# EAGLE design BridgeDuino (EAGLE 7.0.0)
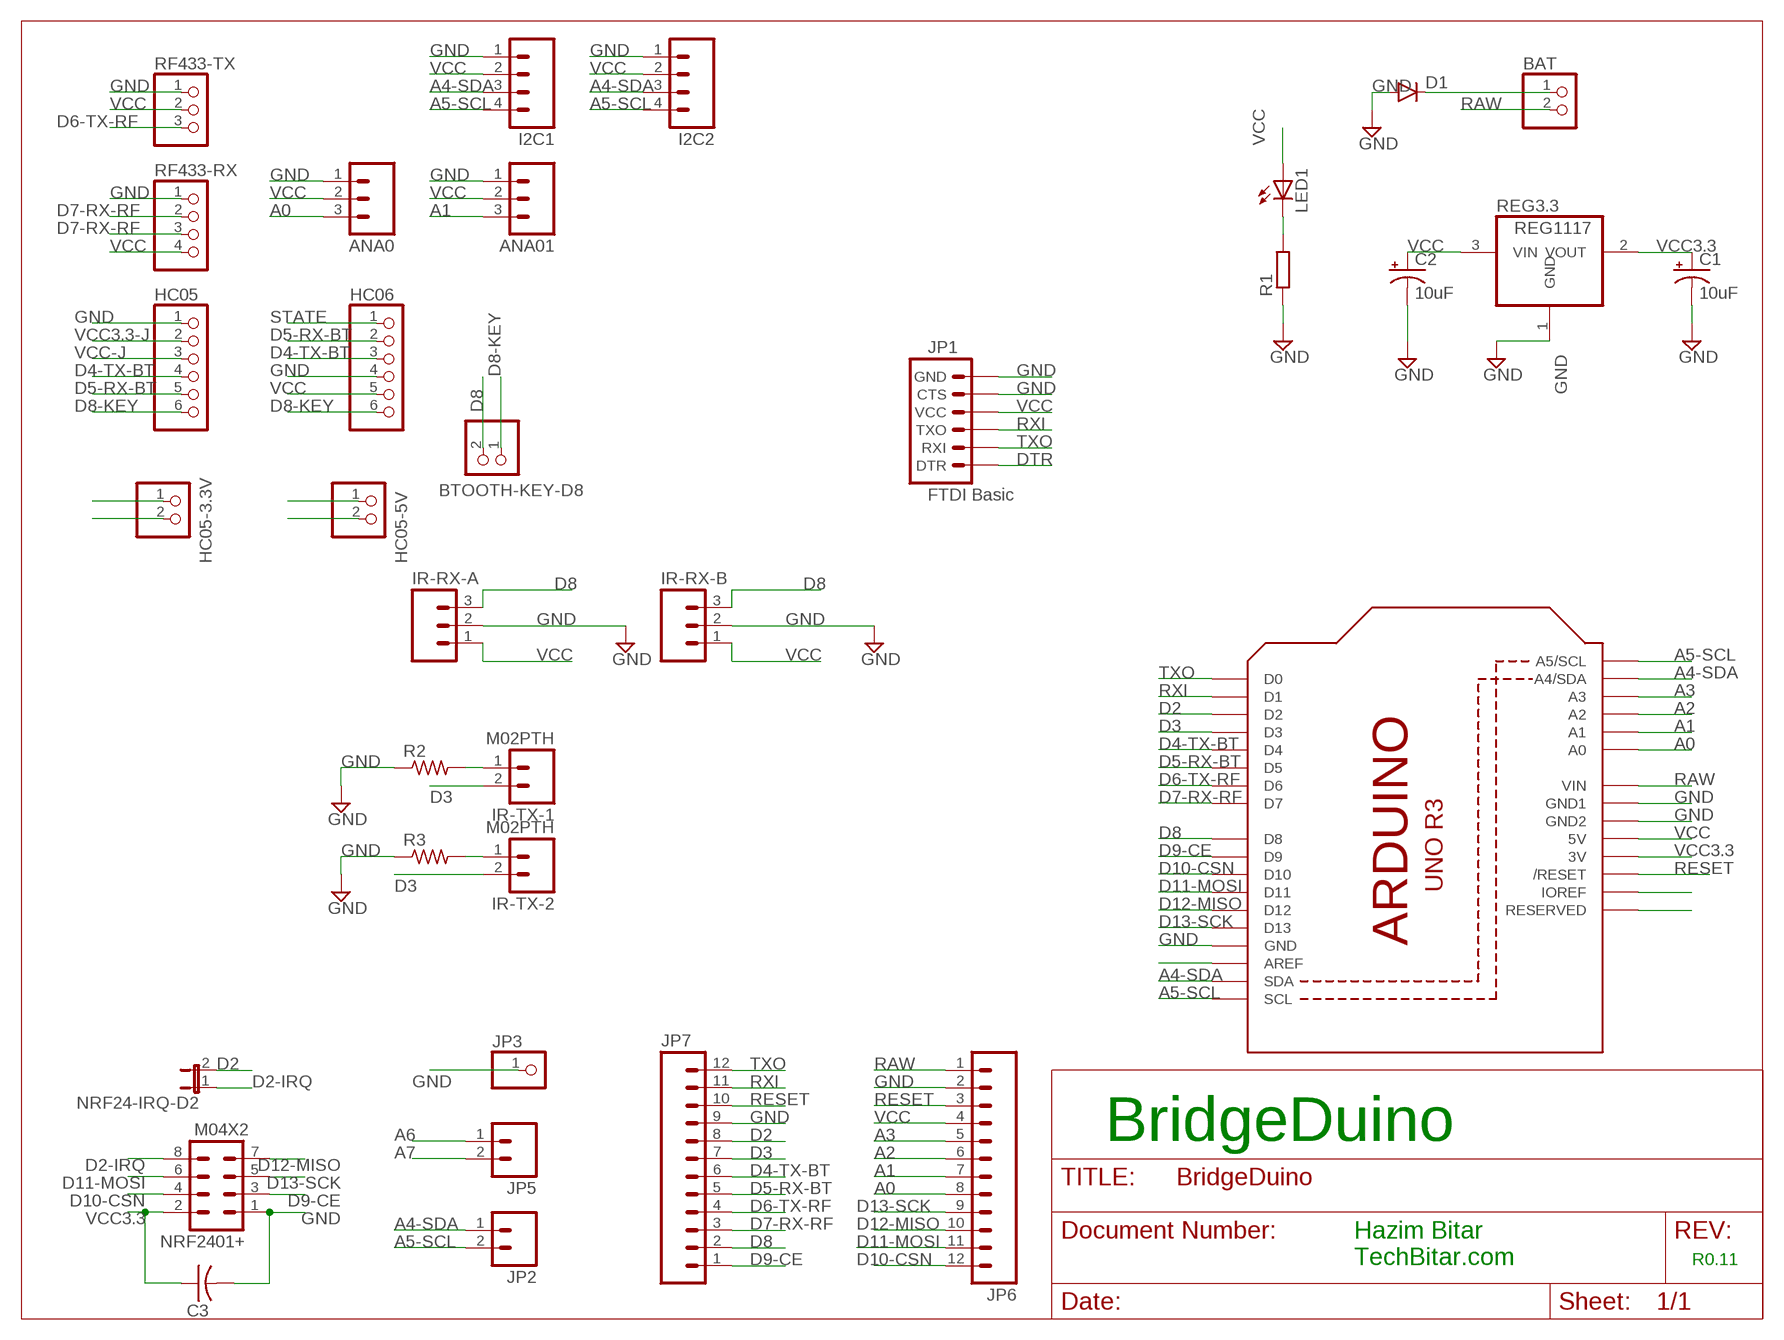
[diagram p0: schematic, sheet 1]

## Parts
ANA0  M03PTH  [1X03]
ANA01  M03PTH  [1X03]
BAT  PINHD-1X2  [1X02]
BTOOTH-KEY-D8  PINHD-1X2  [1X02]
C1  10uF  10UF-16V-10%(TANT)  [EIA3216]
C2  10uF  10UF-16V-10%(TANT)  [EIA3216]
C3  C-US025-024X044  [C025-024X044]
D1  DIODE  [DIODE-1N4001-KIT]
HC05  PINHD-1X6  [1X06]
HC05-3.3V  PINHD-1X2  [1X02]
HC05-5V  PINHD-1X2  [1X02]
HC06  PINHD-1X6  [1X06]
I2C1  M04PTH  [1X04]
I2C2  M04PTH  [1X04]
IR-RX-A  M03PTH  [1X03]
IR-RX-B  M03PTH  [1X03]
IR-TX-1  M02PTH  [1X02]
IR-TX-2  M02PTH  [1X02]
JP1  FTDI Basic  ARDUINO_SERIAL_PROGRAMPTH  [1X06]
JP2  M02PTH  [1X02]
JP3  PINHD-1X1  [1X01]
JP5  M02PTH  [1X02]
JP6  M12PTH  [1X12]
JP7  M12PTH  [1X12]
LED1  LED3MM  [LED3MM]
NRF24-IRQ-D2  JUMPER-2PTH  [1X02]
NRF2401+  M04X2  [2X4]
R1  R-EU_0204/5  [0204/5]
R2  R-US_0204/2V  [0204V]
R3  R-US_0204/2V  [0204V]
REG3.3  REG1117  [SOT223]
RF433-RX  PINHD-1X4  [1X04]
RF433-TX  PINHD-1X3  [1X03]
U1  ARDUINOR3-DIMENSION  [ARDUINOR3]

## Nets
A0 [vcc]: ANA0.3 JP6.8 U1.A0
A1 [vcc]: ANA01.3 JP6.7 U1.A1
A2 [vcc]: JP6.6 U1.A2
A3 [vcc]: JP6.5 U1.A3
A4-SDA [vcc]: I2C1.3 I2C2.3 JP2.1 U1.A4(A4/SDA) U1.SDA
A5-SCL [vcc]: I2C1.4 I2C2.4 JP2.2 U1.A5(A5/SCL) U1.SCL
A6 [vcc]: JP5.1
A7 [vcc]: JP5.2
D2 [vcc]: JP7.8 NRF24-IRQ-D2.2 U1.D2
D2-IRQ [vcc]: NRF24-IRQ-D2.1 NRF2401+.8
D3 [vcc]: IR-TX-1.2 IR-TX-2.2 JP7.7 U1.D3
D4-TX-BT [vcc]: HC05.4 HC06.3 JP7.6 U1.D4
D5-RX-BT [vcc]: HC05.5 HC06.2 JP7.5 U1.D5
D6-TX-RF [vcc]: JP7.4 RF433-TX.3 U1.D6
D7-RX-RF [vcc]: JP7.3 RF433-RX.2 RF433-RX.3 U1.D7
D8 [vcc]: BTOOTH-KEY-D8.2 IR-RX-A.3 IR-RX-B.3 JP7.2 U1.D8
D8-KEY [vcc]: BTOOTH-KEY-D8.1 HC05.6 HC06.6
D9-CE [vcc]: JP7.1 NRF2401+.3 U1.D9
D10-CSN [vcc]: JP6.12 NRF2401+.4 U1.D10
D11-MOSI: JP6.11 NRF2401+.6 U1.D11
D12-MISO [vcc]: JP6.10 NRF2401+.7 U1.D12
D13-SCK [vcc]: JP6.9 NRF2401+.5 U1.D13
DTR: JP1.1(DTR)
GND [vcc]: ANA0.1 ANA01.1 C1.C(-) C2.C(-) C3.2 D1.A HC05.1 HC06.4 I2C1.1 I2C2.1 IR-RX-A.2 IR-RX-B.2 JP1.5(CTS) JP1.6(GND) JP3.1 JP6.2 JP7.9 NRF2401+.1 R1.1 R2.1 R3.1 REG3.3.1(GND) RF433-RX.1 RF433-TX.1 U1.GND U1.GND1 U1.GND2
N$1: BAT.1 D1.C
N$2: IR-TX-2.1 R3.2
N$3: LED1.K(C) R1.2
N$4: IR-TX-1.1 R2.2
N$7 [vcc]: U1.IOREF
N$8 [vcc]: U1.RESERVED
N$24 [vcc]: U1.AREF
RAW [vcc]: BAT.2 JP6.1 U1.VIN
RESET [vcc]: JP6.3 JP7.10 U1.RESET(/RESET)
RXI [vcc]: JP1.3(TXO) JP7.11 U1.D1
STATE [vcc]: HC06.1
TXO [vcc]: JP1.2(RXI) JP7.12 U1.D0
VCC [vcc]: ANA0.2 ANA01.2 C2.A(+) HC05-5V.2 HC06.5 I2C1.2 I2C2.2 IR-RX-A.1 IR-RX-B.1 JP1.4(VCC) JP6.4 LED1.A REG3.3.3(VIN) RF433-RX.4 RF433-TX.2 U1.5V
VCC3.3 [vcc]: C1.A(+) C3.1 HC05-3.3V.2 NRF2401+.2 REG3.3.2(VOUT) U1.3V
VCC3.3-J [vcc]: HC05-3.3V.1 HC05.2
VCC-J [vcc]: HC05-5V.1 HC05.3

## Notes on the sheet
- BridgeDuino
- Hazim Bitar
  TechBitar.com
- R0.11

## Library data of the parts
ANA0 ANA01 IR-RX-A IR-RX-B = SparkFun-Connectors:M03: Header 3 Standard 3-pin 0.1" header. Use with straight break away headers (SKU : PRT-00116), right angle break away headers (PRT-00553), swiss pins (PRT-00743), machine pins (PRT-00117), and female headers (PRT-00115). Molex polarized connector foot print use with SKU : PRT-08232 with associated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
BAT BTOOTH-KEY-D8 HC05-3.3V HC05-5V = pinhead:PINHD-1X2: PIN HEADER
C1 C2 = SparkFun-Capacitors:10UF-16V-10%(TANT): CAP-00811; PROD_ID: CAP-00811
C3 = adafruit:C-US: CAPACITOR, American symbol
D1 = SparkFun-DiscreteSemi:DIODE: Diode
HC05 HC06 = adafruit:PINHD-1X6: PIN HEADER
I2C1 I2C2 = SparkFun-Connectors:M04: Header 4 Standard 4-pin 0.1" header. Use with straight break away headers (SKU : PRT-00116), right angle break away headers (PRT-00553), swiss pins (PRT-00743), machine pins (PRT-00117), and female headers (PRT-00115). Molex polarized connector foot print use with SKU : PRT-08231 with associated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
IR-TX-1 IR-TX-2 = SparkFun-Connectors:M02: Standard 2-pin 0.1" header. Use with
JP1 = SparkFun:ARDUINO_SERIAL_PROGRAM
JP2 JP5 = SparkFun:M02: Header 2
JP3 = adafruit:PINHD-1X1: Pin header 1x1 for 0.1" spacing
JP6 JP7 = SparkFun:M12: Header 12 Standard 12-pin 0.1" header. Use with straight break away headers (SKU : PRT-00116), right angle break away headers (PRT-00553), swiss pins (PRT-00743), machine pins (PRT-00117), and female headers (PRT-00115).
LED1 = led:LED: LED
NRF24-IRQ-D2 = SparkFun-Retired:JUMPER-2: Jumper
NRF2401+ = SparkFun-Connectors:M04X2: .1" header, two rows of four.
R1 = resistor:R-EU_: RESISTOR, European symbol
R2 R3 = adafruit:R-US_: RESISTOR, American symbol
REG3.3 = burr-brown:REG1117: 800mA and 1A Low Dropout (LDO) Positive Regulator 1.8V, 2.5V, 2.85V, 3.3V, 5V, and Adj; MPN: REG1117; OC_FARNELL: 1097566; OC_NEWARK: 14P6981
RF433-RX = pinhead:PINHD-1X4: PIN HEADER
RF433-TX = pinhead:PINHD-1X3: PIN HEADER
U1 = adafruit:ARDUINOR3: This is a new object for the new Arduino R3 - with extra pins that you may want to use (such as IOref, and duplicated A4/A5

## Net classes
0 default: width 0.203 mm
1 vcc: width 0.203 mm

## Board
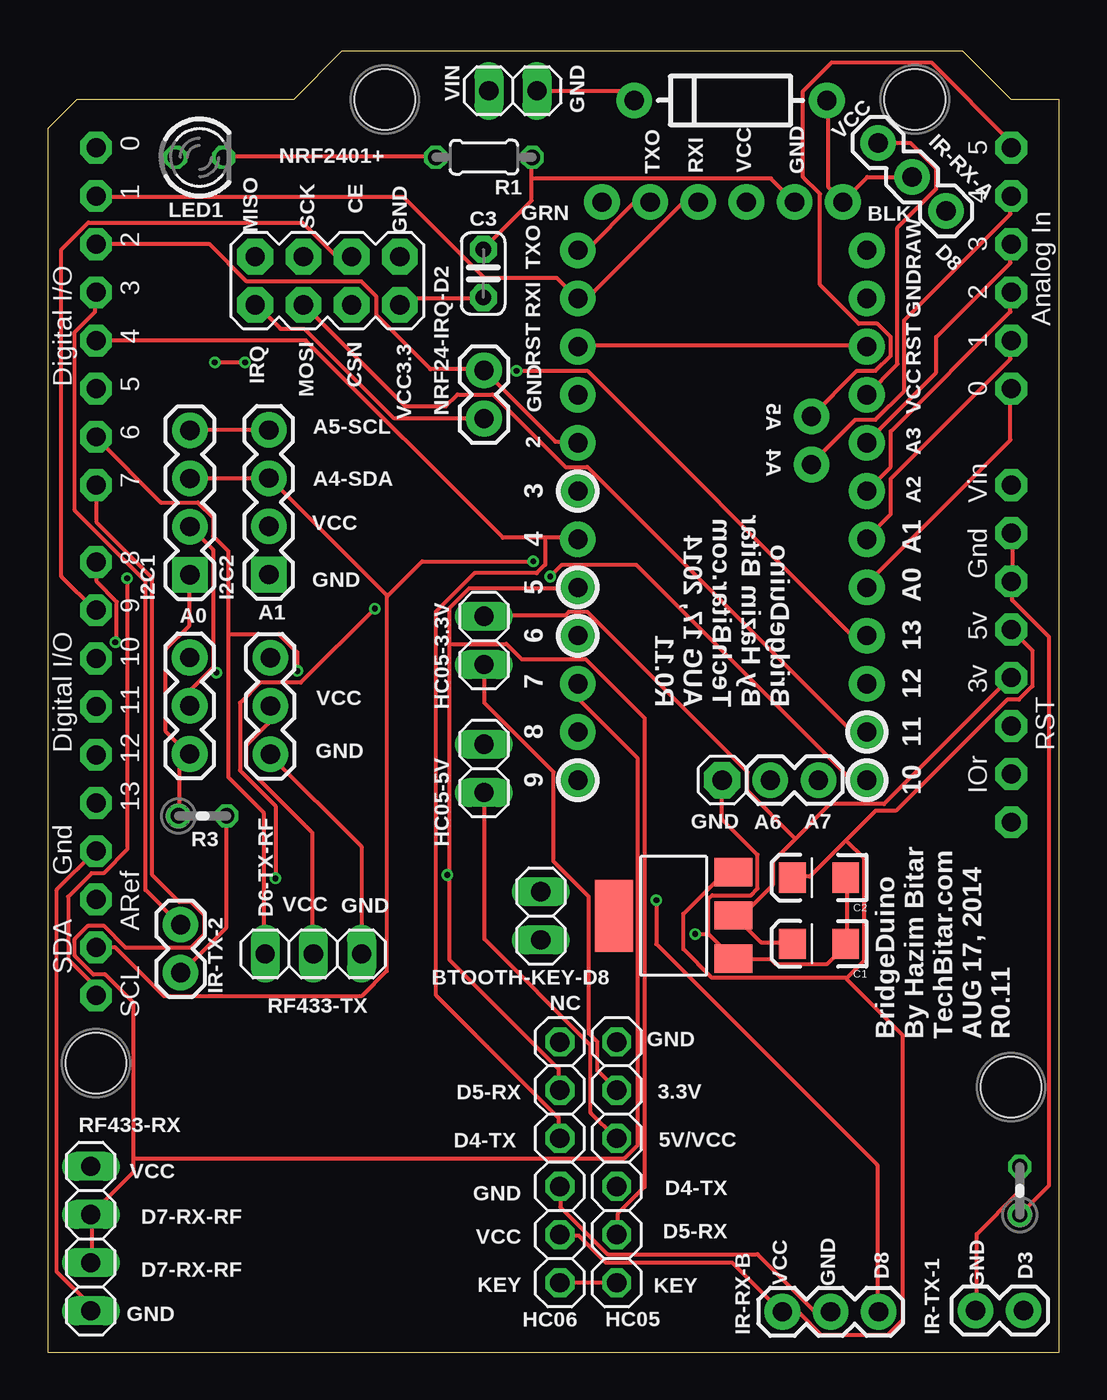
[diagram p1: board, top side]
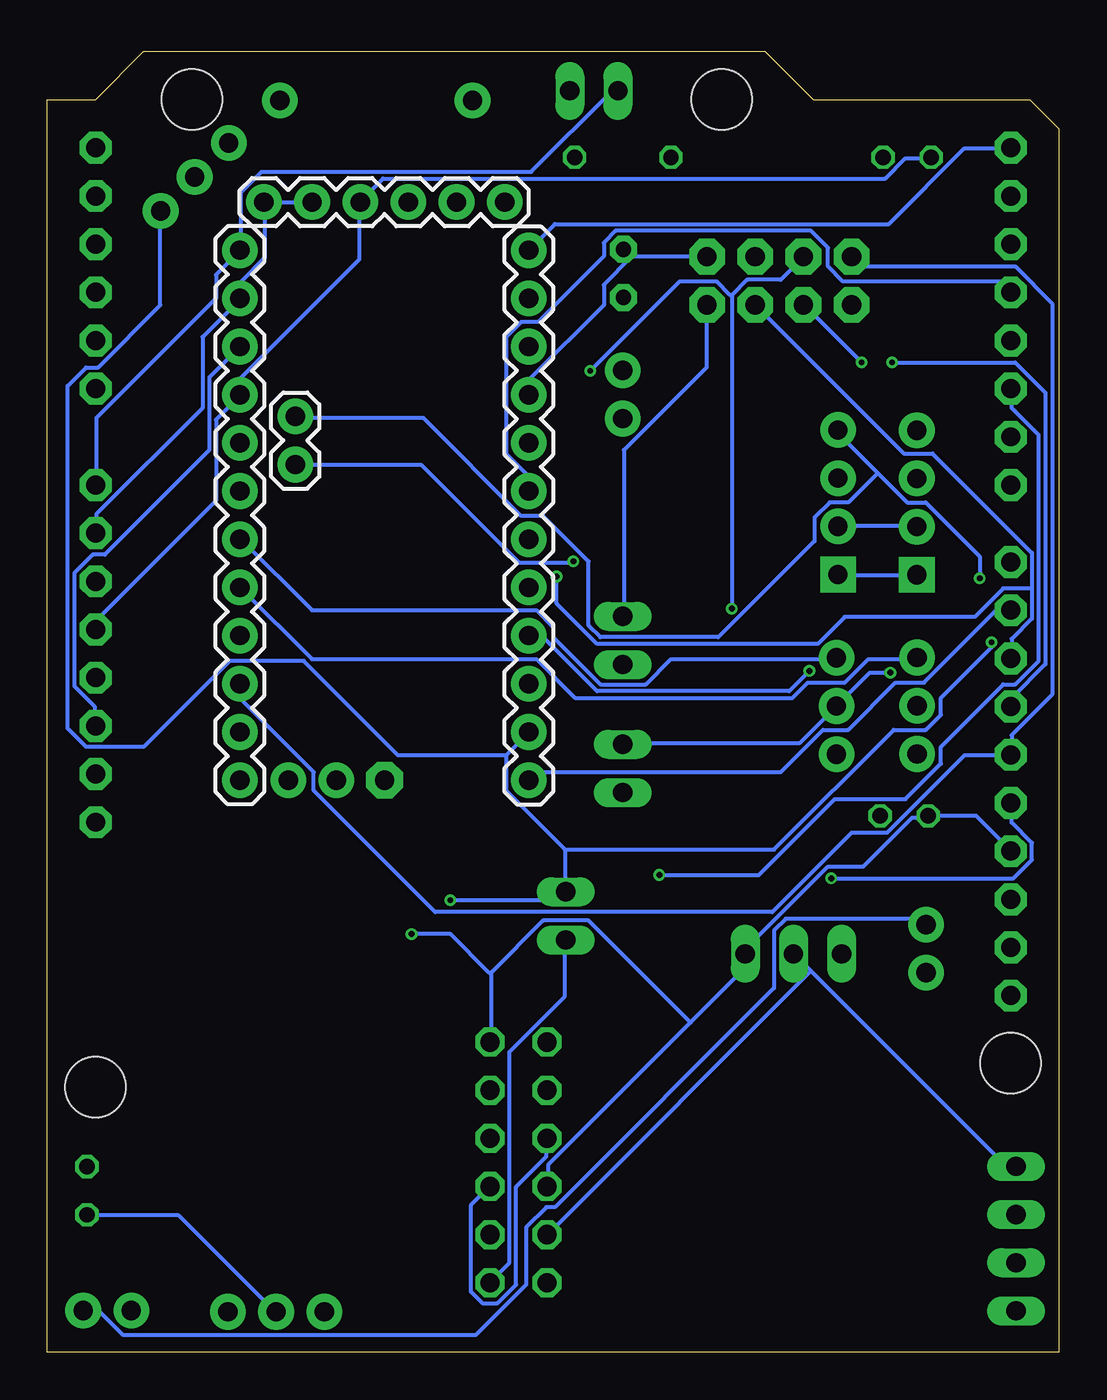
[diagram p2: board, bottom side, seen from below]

Size 53.34 x 68.58 mm. Coordinates in mm from the lower left corner, seen from the top.
Copper layers (1*2*15*16): Top 0.035mm / dielectric 0.2mm / Route2 0.0175mm / dielectric 1.1mm / Route15 0.0175mm / dielectric 0.2mm / Bottom 0.035mm
Design rules "SeeedStudio_DRU_no_angle_20130527 *": minimum track width 6mil, minimum drill 12mil, track to track 6mil, track to pad 6mil, pad to pad 6mil, via to via 6mil, smd to smd 0mil, copper to edge 10mil, drill to drill 10mil, minimum pad ring 6mil, minimum via ring 6mil, stop-mask expansion 2mil, vias tented up to drill 25mil, thermal gap 10mil
Holes 3.2 mm at 2.54,15.24 17.78,66.04 45.72,66.04 50.8,13.97

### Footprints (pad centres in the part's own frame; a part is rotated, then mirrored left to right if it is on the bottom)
1X03 = drill 1.016 pad 1.88: 1 0,0; 2 2.54,0; 3 5.08,0
1X02 = drill 1.016 long: 1 -1.27,0; 2 1.27,0
EIA3216 = smd 1.4 x 1.6: A 1.4,0; C -1.4,0
C025-024X044 = drill 0.813 pad 1.422 octagon: 1 -1.27,0; 2 1.27,0
DIODE-1N4001-KIT = drill 1.016 pad 1.88: A -5.08,0; C 5.08,0
1X06 = drill 1.016 octagon: 1 -6.35,0; 2 -3.81,0; 3 -1.27,0; 4 1.27,0; 5 3.81,0; 6 6.35,0
1X04 = drill 1.016 pad 1.88 square: 1 0,0 | drill 1.016 pad 1.88: 2 2.54,0; 3 5.08,0; 4 7.62,0
1X02' = drill 1.016 pad 1.88: 1 0,0; 2 2.54,0
1X06' = drill 1.016 pad 1.88: 1 0,0; 2 2.54,0; 3 5.08,0; 4 7.62,0; 5 10.16,0; 6 12.7,0
1X01 = drill 1.016 pad 1.93 octagon: 1 0,0
1X12 = drill 1.016 pad 1.88: 1 0,0; 2 2.54,0; 3 5.08,0; 4 7.62,0; 5 10.16,0; 6 12.7,0; 7 15.24,0; 8 17.78,0; 9 20.32,0; 10 22.86,0; 11 25.4,0; 12 27.94,0
LED3MM = drill 0.813 octagon: A -1.27,0; K 1.27,0
2X4 = drill 1.016 pad 1.88 octagon: 1 -3.81,-1.27; 2 -3.81,1.27; 3 -1.27,-1.27; 4 -1.27,1.27; 5 1.27,-1.27; 6 1.27,1.27; 7 3.81,-1.27; 8 3.81,1.27
0204/5 = drill 0.813 octagon: 1 -2.54,0; 2 2.54,0
0204V = drill 0.813 octagon: 1 -1.27,0; 2 1.27,0
SOT223 = smd 1.499 x 2.007: 1 -2.261,-3.15; 2 0.025,-3.15; 3 2.311,-3.15 | smd 3.81 x 2.007: 4 0,3.15
1X04' = drill 1.016 long: 1 -3.81,0; 2 -1.27,0; 3 1.27,0; 4 3.81,0
1X03' = drill 1.016 long: 1 -2.54,0; 2 0,0; 3 2.54,0
ARDUINOR3 = drill 1 pad 1.676 octagon: 3V 35.56,2.54; 5V 38.1,2.54; A0 50.8,2.54; A1 53.34,2.54; A2 55.88,2.54; A3 58.42,2.54; A4 60.96,2.54; A5 63.5,2.54; AREF 23.876,50.8; D0 63.5,50.8; D1 60.96,50.8; D2 58.42,50.8; D3 55.88,50.8; D4 53.34,50.8; D5 50.8,50.8; D6 48.26,50.8; D7 45.72,50.8; D8 41.656,50.8; D9 39.116,50.8; D10 36.576,50.8; D11 34.036,50.8; D12 31.496,50.8; D13 28.956,50.8; GND 26.416,50.8; GND1 43.18,2.54; GND2 40.64,2.54; IOREF 30.48,2.54; RESERVED 27.94,2.54; RESET 33.02,2.54; SCL 18.796,50.8; SDA 21.336,50.8; VIN 45.72,2.54

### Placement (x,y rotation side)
ANA0  7.48,31.54 90 top
ANA01  11.73,31.52 90 top
BAT  24.52,66.51 180 top
BTOOTH-KEY-D8  26,23 90 top
C1  40.66,21.52 180 top
C2  40.66,25.02 180 top
C3  22.96,56.87 90 top
D1  36,66 180 top
HC05  30,10 270 top
HC05-3.3V  23,37.52 90 top
HC05-5V  23,30.78 90 top
HC06  27,10 270 top
I2C1  7.49,40.98 90 top
I2C2  11.65,41 90 top
IR-RX-A  43.78,63.76 315 top
IR-RX-B  38.74,2.13 0 top
IR-TX-1  M02PTH  [1X02']  48.92,2.19 0 top
IR-TX-2  M02PTH  [1X02']  7,20 90 top
JP1  FTDI Basic  [1X06']  29.22,60.64 180 bottom
JP2  [1X02']  40.27,46.8 90 bottom
JP3  35.56,30.16 0 top
JP5  [1X02']  38.1,30.16 0 top
JP6  43.19,58.1 270 bottom
JP7  27.95,30.16 90 bottom
LED1  8,63 0 top
NRF24-IRQ-D2  [1X02']  23,49.22 90 top
NRF2401+  14.75,56.49 180 top
R1  23,63 180 top
R2  51.25,8.51 90 top
R3  8.16,28.27 0 top
REG3.3  33,23 90 top
RF433-RX  [1X04']  2.26,5.98 90 top
RF433-TX  [1X03']  14,21 180 top
U1  53.34,0 90 top

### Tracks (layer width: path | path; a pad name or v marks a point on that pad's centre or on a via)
A0
  Top 0.203: U1.A0 50.76,50.76 50.76,48.09 43.2,40.54 43.2,40.36 JP6.8
  Bottom 0.203: ANA0.3 7.56,36.54 10.05,36.54 11.29,35.29 13.25,35.29 14.05,34.49 25.51,34.49 27.56,36.54 39.38,36.54 43.12,40.27 JP6.8
A1
  Top 0.203: U1.A1 50.76,53.34 50.76,52.36 44.45,46.05 44.45,44.18 43.2,42.94 JP6.7
  Bottom 0.203: ANA01.3 11.73,36.54 20.45,36.54 21.78,35.2 24.18,35.2 26.67,37.69 26.67,38.23 27.56,39.12 39.38,39.12 43.12,42.85 JP6.7
A2
  Top 0.203: U1.A2 50.76,55.83 50.76,54.85 44.45,48.54 44.45,46.67 43.2,45.43 JP6.6
A3
  Top 0.203: U1.A3 50.76,58.41 50.76,57.43 46.85,53.52 46.85,51.65 43.2,48.01 JP6.5
A4-SDA  (via drill 0.3)
  Top 0.203: U1.A4 50.76,60.9 50.76,60.01 45.16,54.41 45.16,50.67 43.65,49.16 42.58,49.16 40.27,46.85 JP2.1 | U1.SDA 3.56,21.34 6.13,18.76 16.54,18.76 17.87,20.09 17.87,39.92 | 17.87,39.92 11.73,46.05 I2C2.3 11.56,46.05 7.56,46.05 I2C1.3 | v25.6,41.69 19.74,41.69 17.96,39.92 17.87,39.92
  Bottom 0.203: v25.6,41.69 25.69,41.6 28.45,41.6 33.6,46.76 40.18,46.76 JP2.1
A5-SCL  (via drill 0.3)
  Top 0.203: U1.A5 50.76,63.56 50.76,63.83 46.58,68.01 41.34,68.01 39.83,66.5 39.83,61.96 40.72,61.07 40.72,56.27 42.76,54.23 43.74,54.23 44.45,53.52 44.45,52.54 43.65,51.74 42.67,51.74 JP2.2 | v4.18,40.8 4.18,26.49 2.93,25.25 2.31,25.25 1.07,24 1.07,20.71 2.49,19.29 2.49,18.85 U1.SCL | I2C1.4 7.56,48.63 I2C2.4
  Bottom 0.203: v4.18,40.8 4.18,41.96 7.02,44.81 8,44.81 9.56,46.36 | 9.56,46.36 11.73,48.54 I2C2.4 | 9.56,46.36 11.11,44.81 12.09,44.81 12.89,44.01 12.89,42.76 17.96,37.69 24.18,37.69 24.8,38.32 24.8,41.69 27.2,44.09 28.36,44.09 33.52,49.25 40.18,49.25 JP2.2
D2
  Top 0.203: U1.D2 2.58,58.41 8.53,58.41 10.49,56.45 16.54,56.45 17.34,55.65 17.34,54.67 20.18,51.83 22.94,51.83 NRF24-IRQ-D2.2 23.02,51.74 26.76,48.01 27.91,48.01 JP7.8
D2-IRQ
  Top 0.203: NRF24-IRQ-D2.1 22.94,49.25 18.22,49.25 13.51,53.96 12.27,53.96 11.02,55.21 NRF2401+.8
D3
  Top 0.203: U1.D3 2.49,55.83 2.49,54.85 1.42,53.78 1.42,44.36 5.16,40.63 5.16,24.36 6.93,22.58 IR-TX-2.2
  Bottom 0.203: IR-TX-1.2 51.38,2.13 50.58,2.13 49.34,0.89 30.76,0.89 28.09,3.56 28.09,6.58 27.03,7.64 26.58,7.64 15.02,19.2 15.02,22.23 14.4,22.85 7.29,22.85 7.02,22.58 IR-TX-2.2 | U1.D3 3.11,56.45 11.38,56.45 12.18,57.25 12.18,58.23 13.07,59.12 23.38,59.12 24,58.5 24,57.78 27.47,54.32 28.36,54.32 29.16,53.52 29.16,47.38 28,46.23 28,45.43 JP7.7
D4-TX-BT
  Top 0.203: U1.D4 13.6,53.34 24,42.94 26.23,42.94 | 26.23,42.94 27.91,42.94 JP7.6 | 26.23,42.94 26.23,41.52 25.78,41.07 22.49,41.07 20.45,39.03 20.45,18.85 26.94,12.36 26.94,11.29 HC06.3
  Bottom 0.203: HC06.3 27.03,11.2 27.03,10.31 28.63,8.71 28.63,3.56 29.6,2.58 30.4,2.58 31.03,3.2 31.03,7.73 30.05,8.71 HC05.4
D5-RX-BT  (via drill 0.3)
  Top 0.203: 21.16,37.34 21.16,39.2 22.23,40.27 27.91,40.27 JP7.5 | 21.16,37.34 21.16,25.16 | 21.16,25.16 21.16,20.71 26.94,14.94 26.94,13.87 HC06.2 | 21.16,37.34 24.18,37.34 24.98,36.54 28.36,36.54 31.47,33.43 31.47,8.71 30.05,7.29 30.05,6.22 HC05.5 | v21.07,25.16 21.16,25.16
  Bottom 0.203: v21.07,25.16 15.82,25.16 11.82,29.16 8.09,29.16 6.22,31.03 6.22,31.91 2.93,35.2 2.31,35.2 1.07,36.45 1.07,48.36 2.49,49.78 2.49,50.76 U1.D5
D6-TX-RF  (via drill 0.3)
  Top 0.203: 9.51,37.87 9.51,42.23 8.71,43.03 8.71,44.01 7.91,44.81 5.96,44.81 2.58,48.18 U1.D6 | 9.51,37.87 9.51,30.32 11.38,28.45 11.38,21.07 RF433-TX.3 | v13.16,35.92 13.16,36.89 12.18,37.87 9.51,37.87
  Bottom 0.203: v13.16,35.92 14.22,34.85 24.36,34.85 27.2,37.69 27.91,37.69 JP7.4
D7-RX-RF
  Top 0.203: RF433-RX.2 2.31,4.8 2.31,7.2 RF433-RX.3 2.31,7.29 4.53,9.51 4.53,10.22 | 4.53,10.22 4.53,18.4 3.02,19.91 2.4,19.91 1.42,20.89 1.42,21.78 2.13,22.49 2.93,22.49 4.09,21.34 7.56,21.34 8.27,22.05 8.27,23.02 7.56,23.74 6.93,23.74 5.51,25.16 5.51,40.8 2.58,43.74 2.58,45.7 U1.D7 | 4.53,10.22 30.4,10.22 31.11,10.94 31.11,31.29 28,34.4 28,35.2 JP7.3
D8  (via drill 0.3)
  Top 0.203: v3.56,37.43 3.65,37.52 3.65,39.56 2.58,40.63 2.58,41.6 U1.D8 | v32.09,23.82 32.09,21.51 43.74,9.87 43.74,2.13 IR-RX-B.3
  Bottom 0.203: 26.05,26.49 26.05,24.36 BTOOTH-KEY-D8.2 26.05,24.18 26.4,23.82 v32.09,23.82 | 26.05,26.49 29.16,29.6 29.16,31.47 | 29.16,31.47 28,32.63 JP7.2 | v3.56,37.43 3.56,37.16 6.22,34.49 6.22,33.6 7.02,32.8 8.71,32.8 15.02,26.49 26.05,26.49 | 29.16,31.47 34.85,31.47 39.83,36.45 43.74,36.45 48.27,31.91 51.3,31.91 52.27,32.89 52.27,50.94 51.3,51.92 50.67,51.92 47.38,55.21 47.38,60.1 IR-RX-A.3
D8-KEY
  Top 0.203: HC06.6 27.03,3.65 29.96,3.65 HC05.6
  Bottom 0.203: BTOOTH-KEY-D8.1 26.05,21.69 26.05,18.76 28.98,15.82 28.98,4.71 29.96,3.73 HC05.6
D9-CE
  Top 0.203: NRF2401+.3 16,57.78 15.2,57.78 13.42,59.56 2.13,59.56 0.71,58.14 0.71,40.89 2.49,39.12 U1.D9
  Bottom 0.203: U1.D9 3.29,39.12 7.11,35.29 8.62,35.29 11.11,32.8 12.45,32.8 14.67,30.58 27.56,30.58 27.91,30.23 JP7.1
D10-CSN  (via drill 0.3)
  Top 0.203: v26.49,40.89 27.11,41.52 31.03,41.52 42.32,30.23 43.12,30.23 JP6.12
  Bottom 0.203: 1.42,40.27 1.42,42.14 6.67,47.38 8.18,47.38 16,55.21 NRF2401+.4 | 1.42,40.27 1.42,38.67 2.49,37.6 2.49,36.63 U1.D10 | v26.49,40.89 26.49,39.47 24.36,37.34 12.71,37.34 11.29,38.76 4.45,38.76 2.93,40.27 1.42,40.27
D11-MOSI  (via drill 0.3)
  Top 0.203: v10.4,52.18 v8.8,52.18 | JP6.11 43.12,32.72 42.41,32.72 28.45,46.67 27.29,46.67 23.47,50.49 21.6,50.49 20.98,49.87 18.85,49.87 13.51,55.21 NRF2401+.6
  Bottom 0.203: v8.8,52.18 2.31,52.18 0.71,50.58 0.71,36.27 2.49,34.49 2.49,34.05 U1.D11 | v10.4,52.18 13.42,55.21 NRF2401+.6
D12-MISO
  Bottom 0.203: NRF2401+.7 10.94,57.7 10.49,57.25 2.31,57.25 0.36,55.3 0.36,34.67 2.49,32.54 2.49,31.56 U1.D12 2.58,31.47 4.98,31.47 9.07,27.38 10.94,27.38 15.11,23.2 32.89,23.2 39.29,29.6 39.29,30.58 43.12,34.4 43.12,35.2 JP6.10
D13-SCK  (via drill 0.3)
  Top 0.203: v12,24.98 12,28.8 10.13,30.67 10.13,34.23 11.2,35.29 13.34,35.29 v17.25,39.2 | v24.71,51.74 28.45,51.74 42.41,37.78 43.12,37.78 JP6.9
  Bottom 0.203: v12,24.98 2.4,24.98 1.42,25.96 1.42,26.85 2.49,27.91 2.49,28.89 U1.D13 | 17.25,55.74 v17.25,39.2 | 17.25,55.74 16.45,56.54 14.67,56.54 13.51,57.7 NRF2401+.5 | v24.71,51.74 20,56.45 18.05,56.45 17.34,55.74 17.25,55.74
GND  (via drill 0.3)
  Top 0.203: 25.51,61.87 25.51,60.72 23.02,58.23 C3.2 | 25.51,61.87 25.51,62.94 R1.1 | U1.GND1 50.85,43.12 50.85,40.72 U1.GND2 50.85,40.63 50.85,39.65 52.81,37.69 52.81,8.8 51.3,7.29 R2.1 | D1.A 41.16,65.96 41.16,61.43 41.87,60.72 JP1.6 41.96,60.72 43.2,61.96 45.52,61.96 IR-RX-A.2 | 25.51,61.87 38.14,61.87 39.29,60.72 JP1.5 | R3.1 6.93,28.36 6.93,30.94 7.47,31.47 ANA0.1 7.38,31.56 6.22,32.72 6.22,37.07 7.47,38.32 7.47,40.98 I2C1.1 | RF433-RX.1 2.22,2.22 2.22,2.49 0.45,4.27 0.45,24.36 2.49,26.4 U1.GND | C2.C 42.14,24.98 42.14,21.6 C1.C 42.05,21.43 41.07,20.45 38.41,20.45 38.14,20.71 36.18,20.71 REG3.3.1 36.09,20.8 34.85,22.05 | JP3.1 35.56,28.09 37.43,26.23 37.43,24.45 37.07,24.09 35.03,24.09 34.85,23.91 34.85,22.05 | RF433-TX.1 16.54,21.07 16.54,26.67 11.73,31.47 ANA01.1 | IR-RX-B.2 41.25,2.13 40.45,2.13 37.43,5.16 29.52,5.16 27.03,7.64 27.03,8.71 HC06.4 | v34.14,22.05 34.85,22.05
  Bottom 0.203: NRF2401+.1 18.58,57.78 22.58,57.78 22.94,58.14 C3.2 22.58,57.7 24,56.27 24,55.21 27.91,51.3 27.91,50.49 JP7.9 | JP1.5 41.87,60.63 JP1.6 41.87,60.54 41.87,57.7 43.12,56.45 43.12,55.56 JP6.2 43.2,55.47 45.16,53.52 45.16,49.78 50.76,44.18 50.76,43.2 U1.GND1 | I2C1.1 7.56,40.98 11.65,40.98 I2C2.1 | U1.GND 2.58,26.49 4.36,28.27 6.84,28.27 R3.1 6.93,28.18 7.73,28.18 10.31,25.6 12.18,25.6 16.54,21.25 16.54,21.07 RF433-TX.1 16.62,20.98 16.62,20.18 19.43,17.38 | R2.1 51.21,7.2 46.41,7.2 41.34,2.13 IR-RX-B.2 | 19.43,17.38 26.94,9.87 26.94,8.8 HC06.4 | 29.96,20 29.96,16.36 HC05.1 | 29.96,20 27.2,22.76 24.8,22.76 19.43,17.38 | v34.14,22.05 32.09,22.05 30.05,20 29.96,20
N$1
  Top 0.203: BAT.1 25.87,66.5 30.4,66.5 30.85,66.05 D1.C
N$2
  Top 0.203: R3.2 9.42,22.4 7.02,20 IR-TX-2.1
N$3
  Top 0.203: LED1.K 9.34,63.03 20.45,63.03 R1.2
N$4
  Top 0.203: R2.2 51.21,9.69 51.21,8.45 48.98,6.22 48.98,2.22 IR-TX-1.1
RAW
  Bottom 0.203: BAT.2 23.29,66.5 23.56,66.5 27.83,62.23 42.05,62.23 43.12,61.16 43.12,58.14 JP6.1 43.2,58.05 44.45,56.81 44.45,55.56 50.76,49.25 50.76,45.78 U1.VIN
RESET
  Top 0.203: JP7.10 28,53.07 43.12,53.07 JP6.3
  Bottom 0.203: U1.RESET 50.85,33.07 50.85,34.05 51.92,35.12 51.92,41.07 50.94,42.05 50.32,42.05 44.81,47.56 44.81,51.38 43.2,52.98 JP6.3
RXI
  Top 0.203: U1.D1 2.58,60.9 18.76,60.9 23.02,56.63 26.85,56.63 27.91,55.56 JP7.11 28,55.65 28.54,55.65 33.52,60.63 34.23,60.63 JP1.3
TXO
  Top 0.203: JP1.2 31.74,60.63 30.94,60.63 28.45,58.14 28,58.14 JP7.12
  Bottom 0.203: U1.D0 2.58,63.48 4.98,63.48 8.98,59.47 26.58,59.47 27.91,58.14 JP7.12
VCC  (via drill 0.3)
  Top 0.203: HC06.5 27.03,6.13 28,6.13 29.43,4.71 36.09,4.71 38.67,2.13 IR-RX-B.1 38.76,2.04 39.65,2.04 40.8,0.89 44.27,0.89 45.07,1.69 45.07,16.71 42.14,19.65 42.14,19.74 | 8.67,36.05 8.71,36.09 8.71,42.32 7.56,43.47 I2C1.2 | 8.67,36.05 7.56,34.94 7.56,34.14 ANA0.2 | ANA01.2 11.65,34.05 11.65,33.16 10.49,32 10.49,30.85 13.96,27.38 13.96,21.07 RF433-TX.2 | v8.89,35.83 8.67,36.05 | 42.09,26.98 43.65,28.54 44.72,28.54 50.58,34.4 51.21,34.4 51.92,35.12 51.92,36.98 U1.5V | 42.09,26.98 40.18,25.07 39.29,25.07 C2.A | 42.14,19.74 35.03,19.74 33.52,21.25 33.52,23.11 35.65,25.25 36.09,25.25 REG3.3.3 | 42.14,19.74 43.03,20.62 43.03,26.05 42.09,26.98 | IR-RX-A.1 43.83,63.74 45.52,63.74 46.85,62.41 46.85,61.34 44.81,59.3 44.81,52.09 43.2,50.49 JP6.4
  Bottom 0.203: I2C2.2 11.65,43.56 7.56,43.56 I2C1.2 | HC05-5V.2 22.94,32.09 13.69,32.09 11.73,34.05 ANA01.2 11.65,34.14 9.96,35.83 v8.89,35.83 | 13.07,20.09 13.96,20.98 RF433-TX.2 | 13.07,20.09 2.85,9.87 2.31,9.87 RF433-RX.4 | 13.07,20.09 26.94,6.22 HC06.5 | LED1.A 6.76,62.94 8.09,62.94 9.16,61.87 35.65,61.87 36.8,60.72 JP1.4 36.89,60.63 36.89,57.61 43.12,51.38 43.12,50.49 JP6.4 43.2,50.41 44.45,49.16 44.45,44.9 50.76,38.58 50.76,38.14 U1.5V
VCC3.3
  Top 0.203: C3.1 22.94,55.56 18.85,55.56 18.58,55.3 NRF2401+.2 | C1.A 39.2,21.6 37.6,21.6 36.18,23.02 REG3.3.2 36.45,22.85 38.23,24.62 38.23,25.87 39.43,27.07 | 39.43,27.07 41.25,28.89 44.09,28.89 50.76,35.56 U1.3V | 39.43,27.07 36.89,29.6 36.89,30.58 28.45,39.03 27.47,39.03 27.29,38.85 23.02,38.85 HC05-3.3V.2
  Bottom 0.203: HC05-3.3V.2 22.94,38.85 22.94,47.56 18.58,51.92 18.58,55.21 NRF2401+.2
VCC3.3-J
  Top 0.203: HC05-3.3V.1 23.02,36.18 23.02,34.23 26.67,30.58 26.67,25.87 28.54,24 28.54,16.8 28.98,16.36 28.98,14.85 29.96,13.87 HC05.2
VCC-J
  Top 0.203: HC05-5V.1 23.02,29.43 23.02,21.78 28.63,16.18 28.63,12.62 29.96,11.29 HC05.3

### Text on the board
tPlace: VIN | GND | VCC | MISO | SCK | CE | GND | TXO | RXI | VCC | GND | GRN | BLK | D8 | TXO | RAW | RXI | GND | IRQ | MOSI | CSN | VCC3.3 | RST | RST | GND | A5 | VCC | A5-SCL | 2 | A3 | A4-SDA | A4 | 3 | A2 | VCC | 4 | A1 | GND | 5 | A0 | A1 | A0 | 6 | 13 | 7 | VCC | BridgeDuino / By Hazim Bitar / TechBitar.com / AUG 17, 2014 / R0.11 | 12 | 8 | 11 | GND | 9 | 10 | GND | A6 | A7 | VCC | GND | D6-TX-RF | NC | GND | BridgeDuino / By Hazim Bitar / TechBitar.com / AUG 17, 2014 / R0.11 | D5-RX | 3.3V | D4-TX | 5V/VCC | VCC | GND | D4-TX | D7-RX-RF | D5-RX | VCC | VCC | GND | GND | D7-RX-RF | D8 | D3 | KEY | KEY | GND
